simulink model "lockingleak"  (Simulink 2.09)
settings: Solver=ode1  StartTime=0.0  StopTime=1  FixedStep=0.001  MaxStep=0.001  RelTol=1e-5  AbsTol=1e-6

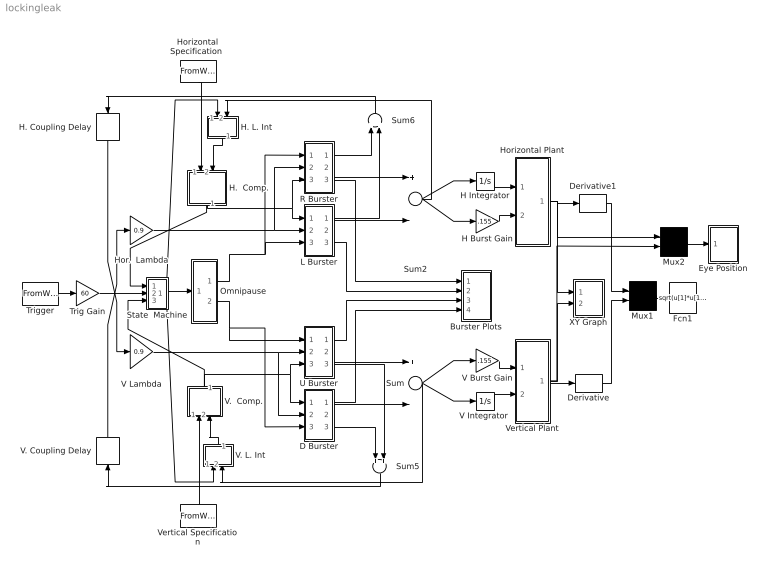
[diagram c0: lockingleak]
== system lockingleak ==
  Burster Plots : Subsystem
  D Burster : Subsystem
  Derivative : Derivative
  Derivative1 : Derivative
  Eye Position : Subsystem  mask(Graph scope.){}
      mask help: Graph scope using MATLAB graph window. Enter plotting ranges and line type.
      mask init:
      | color = @4; ax = [0, @1, @2, @3]; dt = -1;
  Fcn1 : Fcn  Expr=sqrt(u[1]*u[1]+u[2]*u[2])
  H Burst Gain : Gain  Gain=.155
  H Integrator : Integrator  ExternalReset=none  InitialConditionSource=internal  InitialCondition=0  LimitOutput=off  UpperSaturationLimit=inf  LowerSaturationLimit=-inf  ShowSaturationPort=off  ShowStatePort=off  AbsoluteTolerance=auto
  H.  Comp. : Subsystem  Orientation=down
  H. Coupling Delay : TransportDelay  Orientation=down  DelayTime=.001  InitialInput=00  BufferSize=1024
  H. L. Int : Subsystem  Orientation=down
  Hor.  Lambda : Gain  Gain=0.9
  Horizontal Plant : Subsystem
  "Horizontal Specification " : FromWorkspace  Orientation=down  VariableName=hspec
  L Burster : Subsystem
  Mux1 : Mux  Inputs=2
  Mux2 : Mux  Inputs=2
  Omnipause : Subsystem
  R Burster : Subsystem
  State  Machine : Subsystem
  Sum : Sum  Inputs=+-
  Sum2 : Sum  Inputs=+-
  Sum5 : Sum  Orientation=down  Inputs=++
  Sum6 : Sum  Orientation=up  Inputs=++
  Trig Gain : Gain  Gain=60
  Trigger : FromWorkspace  VariableName=trigspec
  U Burster : Subsystem
  V Burst Gain : Gain  Gain=.155
  "V Integrator " : Integrator  ExternalReset=none  InitialConditionSource=internal  InitialCondition=0  LimitOutput=off  UpperSaturationLimit=inf  LowerSaturationLimit=-inf  ShowSaturationPort=off  ShowStatePort=off  AbsoluteTolerance=auto
  V Lambda : Gain  Gain=0.9
  V.  Comp. : Subsystem  Orientation=up
  V. Coupling Delay : TransportDelay  Orientation=up  DelayTime=.001  InitialInput=00  BufferSize=1024
  V. L. Int : Subsystem  Orientation=up
  Vertical Plant : Subsystem
  Vertical Specification : FromWorkspace  Orientation=up  VariableName=vspec
  XY Graph : Subsystem  mask(XY scope.){}
      mask help: XY scope using MATLAB graph window. First input is used as time base. Enter plotting ranges.
      mask init:
      | ax = [@1, @2, @3, @4];st=-1;
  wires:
  State  Machine/1(out_2) -> H. L. Int/1(STATE Input), Omnipause/1(in_1), V. L. Int/1(OPN Input)
  Trig Gain/1 -> State  Machine/2(in_2)
  V.  Comp./1(out_1) -> State  Machine/3(in_3), D Burster/1(in_1), U Burster/3(in_1)
  H.  Comp./1(out_1) -> State  Machine/1(in_1), R Burster/3(in_1), L Burster/1(in_1)
  Omnipause/2(out_4) -> U Burster/1(in_3), D Burster/3(in_3)
  H. L. Int/1(out_1) -> H.  Comp./2(in_2)
  Omnipause/1(out_1) -> R Burster/1(in_3), L Burster/3(in_3)
  Hor.  Lambda/1 -> R Burster/2(in_2), L Burster/2(in_2)
  Mux2/1 -> Eye Position/1(x)
  Horizontal Plant/1(out_1) -> Mux2/1, Derivative1/1, XY Graph/1(x)
  H. Coupling Delay/1 -> V Lambda/1
  V. Coupling Delay/1 -> Hor.  Lambda/1
  Trigger/1 -> Trig Gain/1
  R Burster/1(out_2) -> Sum6/1
  V. L. Int/1(out_1) -> V.  Comp./2(in_5)
  Fcn1/1 -> ?
  Derivative1/1 -> Mux1/1
  Derivative/1 -> Mux1/2
  Mux1/1 -> Fcn1/1
  Vertical Plant/1(out_1) -> Mux2/2, Derivative/1, XY Graph/2(y)
  "Horizontal Specification "/1 -> H.  Comp./1(in_1)
  Vertical Specification/1 -> V.  Comp./1(in_4)
  Sum5/1 -> V. Coupling Delay/1
  Sum6/1 -> H. Coupling Delay/1
  L Burster/1(out_1) -> Sum6/2
  V Lambda/1 -> D Burster/2(in_2), U Burster/2(in_2)
  R Burster/3(out_4) -> Burster Plots/1(in_1)
  L Burster/3(out_3) -> Burster Plots/2(in_2)
  D Burster/1(out_1) -> Burster Plots/4(in_4)
  D Burster/2(out_2) -> Sum/2
  D Burster/3(out_3) -> Sum5/1
  U Burster/1(out_2) -> Burster Plots/3(in_3)
  U Burster/2(out_3) -> Sum/1
  U Burster/3(out_4) -> Sum5/2
  R Burster/2(out_3) -> Sum2/1
  L Burster/2(out_2) -> Sum2/2
  Sum/1 -> V. L. Int/2(BURST Input), "V Integrator "/1, V Burst Gain/1
  "V Integrator "/1 -> Vertical Plant/2(in_2)
  V Burst Gain/1 -> Vertical Plant/1(in_1)
  Sum2/1 -> H. L. Int/2(BURST Input), H Burst Gain/1, H Integrator/1
  H Burst Gain/1 -> Horizontal Plant/2(in_2)
  H Integrator/1 -> Horizontal Plant/1(in_1)

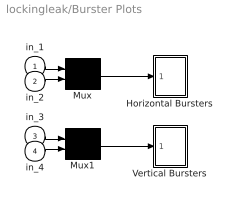
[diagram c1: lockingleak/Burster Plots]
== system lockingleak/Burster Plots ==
  in_1 : Inport  Port=1  PortWidth=-1  SampleTime=-1
  in_2 : Inport  Port=2  PortWidth=-1  SampleTime=-1
  in_3 : Inport  Port=3  PortWidth=-1  SampleTime=-1
  in_4 : Inport  Port=4  PortWidth=-1  SampleTime=-1
  Horizontal Bursters : Subsystem  mask(Graph scope.){}
      mask help: Graph scope using MATLAB graph window. Enter plotting ranges and line type.
      mask init:
      | color = @4; ax = [0, @1, @2, @3]; dt = -1;
  Mux : Mux  Inputs=2
  Mux1 : Mux  Inputs=2
  Vertical Bursters : Subsystem  mask(Graph scope.){}
      mask help: Graph scope using MATLAB graph window. Enter plotting ranges and line type.
      mask init:
      | color = @4; ax = [0, @1, @2, @3]; dt = -1;
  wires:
  in_4/1 -> Mux1/2
  in_3/1 -> Mux1/1
  in_2/1 -> Mux/2
  in_1/1 -> Mux/1
  Mux/1 -> Horizontal Bursters/1(x)
  Mux1/1 -> Vertical Bursters/1(x)

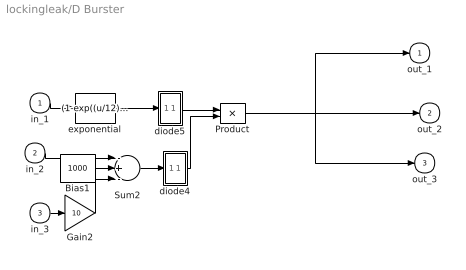
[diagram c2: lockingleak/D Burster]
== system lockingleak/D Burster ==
  in_1 : Inport  Port=1  PortWidth=-1  SampleTime=-1
  in_2 : Inport  Port=2  PortWidth=-1  SampleTime=-1
  in_3 : Inport  Port=3  PortWidth=-1  SampleTime=-1
  Bias1 : Constant  Value=1000
  Gain2 : Gain  Gain=10
  Product : Product  Inputs=2
  Sum2 : Sum  Inputs=-+-
  diode4 : Subsystem
  diode5 : Subsystem
  exponential : Fcn  Expr=(1-exp((u/12)))
  out_1 : Outport  Port=1  InitialOutput=0
  out_2 : Outport  Port=2  InitialOutput=0
  out_3 : Outport  Port=3  InitialOutput=0
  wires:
  in_1/1 -> exponential/1
  Bias1/1 -> Sum2/2
  in_2/1 -> Sum2/1
  in_3/1 -> Gain2/1
  Gain2/1 -> Sum2/3
  Sum2/1 -> diode4/1(in_1)
  diode4/1(out_1) -> Product/2
  exponential/1 -> diode5/1(in_1)
  diode5/1(out_1) -> Product/1
  Product/1 -> out_1/1, out_2/1, out_3/1

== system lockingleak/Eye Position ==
  x : Inport  Port=1  PortWidth=-1  SampleTime=-1
  "S-function M-file which plots lines " : S-Function  FunctionName=sfuny  Parameters=ax, color,dt
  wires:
  x/1 -> "S-function M-file which plots lines "/1

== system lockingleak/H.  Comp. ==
  in_1 : Inport  Port=1  PortWidth=-1  SampleTime=-1
  in_2 : Inport  Port=2  PortWidth=-1  SampleTime=-1
  Sum : Sum  Inputs=+-
  out_1 : Outport  Port=1  InitialOutput=0
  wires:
  in_2/1 -> Sum/2
  in_1/1 -> Sum/1
  Sum/1 -> out_1/1

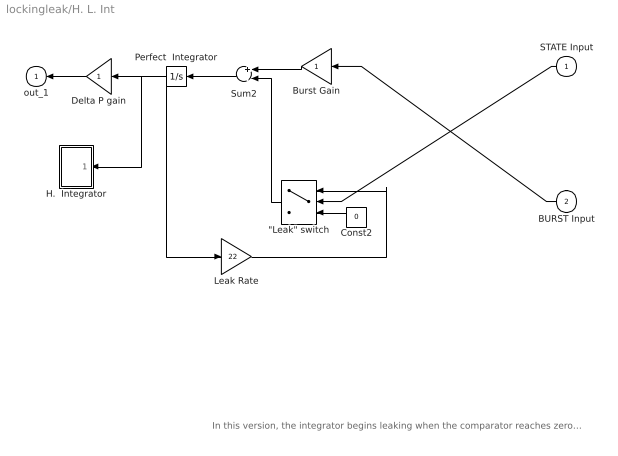
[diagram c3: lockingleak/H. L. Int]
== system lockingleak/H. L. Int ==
  note: In this version, the integrator begins leaking when the comparator reaches zero, and won't stop leaking until either the trigger arrives or the integrator's value goes to zero
  STATE Input : Inport  Orientation=left  Port=1  PortWidth=-1  SampleTime=-1
  BURST Input : Inport  Orientation=left  Port=2  PortWidth=-1  SampleTime=-1
  "\"Leak\" switch" : Switch  Orientation=left  Threshold=0.5
  Burst Gain : Gain  Orientation=left  Gain=1
  Const2 : Constant  Orientation=left  Value=0
  Delta P gain : Gain  Orientation=left  Gain=1
  H.  Integrator : Subsystem  Orientation=left  mask(Graph scope.){}
      mask help: Graph scope using MATLAB graph window. Enter plotting ranges and line type.
      mask init:
      | color = @4; ax = [0, @1, @2, @3]; dt = -1;
  Leak Rate : Gain  Gain=22
  Perfect  Integrator : Integrator  Orientation=left  ExternalReset=none  InitialConditionSource=internal  InitialCondition=0  LimitOutput=off  UpperSaturationLimit=inf  LowerSaturationLimit=-inf  ShowSaturationPort=off  ShowStatePort=off  AbsoluteTolerance=auto
  Sum2 : Sum  Orientation=left  Inputs=+-
  out_1 : Outport  Orientation=left  Port=1  InitialOutput=0
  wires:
  BURST Input/1 -> Burst Gain/1
  STATE Input/1 -> "\"Leak\" switch"/2
  Const2/1 -> "\"Leak\" switch"/3
  "\"Leak\" switch"/1 -> Sum2/2
  Leak Rate/1 -> "\"Leak\" switch"/1
  Perfect  Integrator/1 -> H.  Integrator/1(x), Leak Rate/1, Delta P gain/1
  Burst Gain/1 -> Sum2/1
  Delta P gain/1 -> out_1/1
  Sum2/1 -> Perfect  Integrator/1

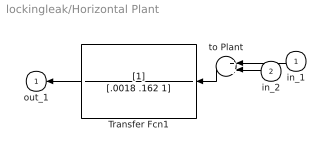
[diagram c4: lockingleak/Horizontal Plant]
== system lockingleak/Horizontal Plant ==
  in_1 : Inport  Orientation=left  Port=1  PortWidth=-1  SampleTime=-1
  in_2 : Inport  Orientation=left  Port=2  PortWidth=-1  SampleTime=-1
  Transfer Fcn1 : TransferFcn  Orientation=left  Numerator=[1]  Denominator=[.0018 .162 1]
  to Plant : Sum  Orientation=left  Inputs=++
  out_1 : Outport  Orientation=left  Port=1  InitialOutput=0
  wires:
  Transfer Fcn1/1 -> out_1/1
  in_2/1 -> to Plant/2
  in_1/1 -> to Plant/1
  to Plant/1 -> Transfer Fcn1/1

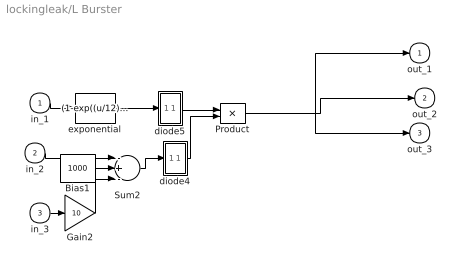
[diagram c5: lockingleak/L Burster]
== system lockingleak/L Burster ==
  in_1 : Inport  Port=1  PortWidth=-1  SampleTime=-1
  in_2 : Inport  Port=2  PortWidth=-1  SampleTime=-1
  in_3 : Inport  Port=3  PortWidth=-1  SampleTime=-1
  Bias1 : Constant  Value=1000
  Gain2 : Gain  Gain=10
  Product : Product  Inputs=2
  Sum2 : Sum  Inputs=-+-
  diode4 : Subsystem
  diode5 : Subsystem
  exponential : Fcn  Expr=(1-exp((u/12)))
  out_1 : Outport  Port=1  InitialOutput=0
  out_2 : Outport  Port=2  InitialOutput=0
  out_3 : Outport  Port=3  InitialOutput=0
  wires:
  Product/1 -> out_3/1, out_2/1, out_1/1
  diode5/1(out_1) -> Product/1
  exponential/1 -> diode5/1(in_1)
  diode4/1(out_1) -> Product/2
  Sum2/1 -> diode4/1(in_1)
  Gain2/1 -> Sum2/3
  in_3/1 -> Gain2/1
  in_2/1 -> Sum2/1
  Bias1/1 -> Sum2/2
  in_1/1 -> exponential/1

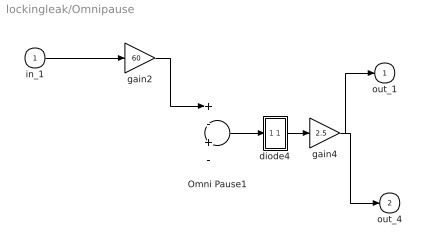
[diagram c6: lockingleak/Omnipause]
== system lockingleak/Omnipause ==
  in_1 : Inport  Port=1  PortWidth=-1  SampleTime=-1
  Omni Pause1 : Sum  Inputs=+-+-
  diode4 : Subsystem
  gain2 : Gain  Gain=60
  gain4 : Gain  Gain=2.5
  out_1 : Outport  Port=1  InitialOutput=0
  out_4 : Outport  Port=2  InitialOutput=0
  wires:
  in_1/1 -> gain2/1
  gain4/1 -> out_4/1, out_1/1
  diode4/1(out_1) -> gain4/1
  gain2/1 -> Omni Pause1/1
  Omni Pause1/1 -> diode4/1(in_1)

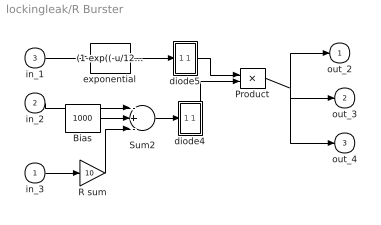
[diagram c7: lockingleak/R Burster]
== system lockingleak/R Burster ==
  in_3 : Inport  Port=1  PortWidth=-1  SampleTime=-1
  in_2 : Inport  Port=2  PortWidth=-1  SampleTime=-1
  in_1 : Inport  Port=3  PortWidth=-1  SampleTime=-1
  Bias : Constant  Value=1000
  Product : Product  Inputs=2
  R sum : Gain  Gain=10
  Sum2 : Sum  Inputs=-+-
  diode4 : Subsystem
  diode5 : Subsystem
  exponential : Fcn  Expr=(1-exp((-u/12)))
  out_2 : Outport  Port=1  InitialOutput=0
  out_3 : Outport  Port=2  InitialOutput=0
  out_4 : Outport  Port=3  InitialOutput=0
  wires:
  diode5/1(out_1) -> Product/1
  exponential/1 -> diode5/1(in_1)
  diode4/1(out_1) -> Product/2
  Sum2/1 -> diode4/1(in_1)
  in_1/1 -> exponential/1
  in_2/1 -> Sum2/1
  Bias/1 -> Sum2/2
  Product/1 -> out_2/1, out_4/1, out_3/1
  in_3/1 -> R sum/1
  R sum/1 -> Sum2/3

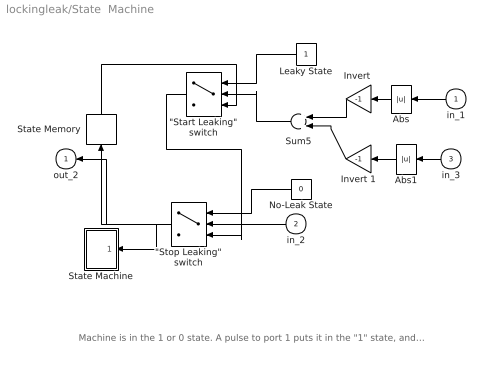
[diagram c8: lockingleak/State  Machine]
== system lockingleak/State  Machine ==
  note: Machine is in the 1 or 0 state. A pulse to port 1 puts it in the "1" state, and a pulse to port 2 puts it in the "0" state.
  in_1 : Inport  Orientation=left  Port=1  PortWidth=-1  SampleTime=-1
  in_2 : Inport  Orientation=left  Port=2  PortWidth=-1  SampleTime=-1
  in_3 : Inport  Orientation=left  Port=3  PortWidth=-1  SampleTime=-1
  "\"Start Leaking\" switch" : Switch  Orientation=left  Threshold=-2
  "\"Stop Leaking\" switch" : Switch  Orientation=left  Threshold=0.001
  Abs : Abs  Orientation=left
  Abs1 : Abs  Orientation=left
  "Invert " : Gain  Orientation=left  Gain=-1
  Invert 1 : Gain  Orientation=left  Gain=-1
  Leaky State : Constant  Orientation=left  Value=1
  No-Leak State : Constant  Orientation=left  Value=0
  State Memory : Memory  Orientation=up  X0=0  InheritSampleTime=off
  State Machine : Subsystem  Orientation=left  mask(Graph scope.){}
      mask help: Graph scope using MATLAB graph window. Enter plotting ranges and line type.
      mask init:
      | color = @4; ax = [0, @1, @2, @3]; dt = -1;
  Sum5 : Sum  Orientation=left  Inputs=++
  out_2 : Outport  Orientation=left  Port=1  InitialOutput=0
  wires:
  Sum5/1 -> "\"Start Leaking\" switch"/2
  "Invert "/1 -> Sum5/1
  Invert 1/1 -> Sum5/2
  Abs1/1 -> Invert 1/1
  in_3/1 -> Abs1/1
  No-Leak State/1 -> "\"Stop Leaking\" switch"/1
  "\"Start Leaking\" switch"/1 -> "\"Stop Leaking\" switch"/3
  Leaky State/1 -> "\"Start Leaking\" switch"/1
  State Memory/1 -> "\"Start Leaking\" switch"/3
  Abs/1 -> "Invert "/1
  "\"Stop Leaking\" switch"/1 -> State Machine/1(x), State Memory/1, out_2/1
  in_1/1 -> Abs/1
  in_2/1 -> "\"Stop Leaking\" switch"/2

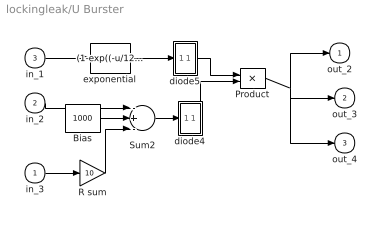
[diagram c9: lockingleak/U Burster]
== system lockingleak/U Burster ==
  in_3 : Inport  Port=1  PortWidth=-1  SampleTime=-1
  in_2 : Inport  Port=2  PortWidth=-1  SampleTime=-1
  in_1 : Inport  Port=3  PortWidth=-1  SampleTime=-1
  Bias : Constant  Value=1000
  Product : Product  Inputs=2
  R sum : Gain  Gain=10
  Sum2 : Sum  Inputs=-+-
  diode4 : Subsystem
  diode5 : Subsystem
  exponential : Fcn  Expr=(1-exp((-u/12)))
  out_2 : Outport  Port=1  InitialOutput=0
  out_3 : Outport  Port=2  InitialOutput=0
  out_4 : Outport  Port=3  InitialOutput=0
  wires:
  diode5/1(out_1) -> Product/1
  exponential/1 -> diode5/1(in_1)
  diode4/1(out_1) -> Product/2
  Sum2/1 -> diode4/1(in_1)
  in_1/1 -> exponential/1
  in_2/1 -> Sum2/1
  Bias/1 -> Sum2/2
  Product/1 -> out_2/1, out_4/1, out_3/1
  in_3/1 -> R sum/1
  R sum/1 -> Sum2/3

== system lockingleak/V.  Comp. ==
  in_4 : Inport  Port=1  PortWidth=-1  SampleTime=-1
  in_5 : Inport  Port=2  PortWidth=-1  SampleTime=-1
  Sum : Sum  Inputs=-+
  out_1 : Outport  Port=1  InitialOutput=0
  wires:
  in_4/1 -> Sum/2
  in_5/1 -> Sum/1
  Sum/1 -> out_1/1

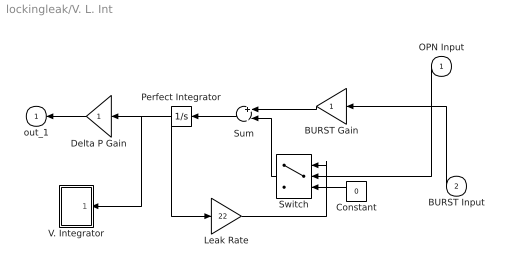
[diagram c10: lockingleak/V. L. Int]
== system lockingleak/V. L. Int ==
  OPN Input : Inport  Orientation=left  Port=1  PortWidth=-1  SampleTime=-1
  BURST Input : Inport  Orientation=left  Port=2  PortWidth=-1  SampleTime=-1
  BURST Gain : Gain  Orientation=left  Gain=1
  Constant : Constant  Orientation=left  Value=0
  Delta P Gain : Gain  Orientation=left  Gain=1
  Leak Rate : Gain  Gain=22
  Perfect Integrator : Integrator  Orientation=left  ExternalReset=none  InitialConditionSource=internal  InitialCondition=0  LimitOutput=off  UpperSaturationLimit=inf  LowerSaturationLimit=-inf  ShowSaturationPort=off  ShowStatePort=off  AbsoluteTolerance=auto
  Sum : Sum  Orientation=left  Inputs=+-
  Switch : Switch  Orientation=left  Threshold=0.5
  V. Integrator : Subsystem  Orientation=left  mask(Graph scope.){}
      mask help: Graph scope using MATLAB graph window. Enter plotting ranges and line type.
      mask init:
      | color = @4; ax = [0, @1, @2, @3]; dt = -1;
  out_1 : Outport  Orientation=left  Port=1  InitialOutput=0
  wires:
  BURST Input/1 -> BURST Gain/1
  OPN Input/1 -> Switch/2
  Sum/1 -> Perfect Integrator/1
  Delta P Gain/1 -> out_1/1
  BURST Gain/1 -> Sum/1
  Perfect Integrator/1 -> Delta P Gain/1, Leak Rate/1, V. Integrator/1(x)
  Leak Rate/1 -> Switch/1
  Constant/1 -> Switch/3
  Switch/1 -> Sum/2

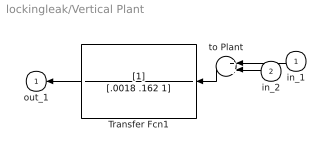
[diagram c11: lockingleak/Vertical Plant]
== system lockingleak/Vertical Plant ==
  in_1 : Inport  Orientation=left  Port=1  PortWidth=-1  SampleTime=-1
  in_2 : Inport  Orientation=left  Port=2  PortWidth=-1  SampleTime=-1
  Transfer Fcn1 : TransferFcn  Orientation=left  Numerator=[1]  Denominator=[.0018 .162 1]
  to Plant : Sum  Orientation=left  Inputs=++
  out_1 : Outport  Orientation=left  Port=1  InitialOutput=0
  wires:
  Transfer Fcn1/1 -> out_1/1
  in_2/1 -> to Plant/2
  in_1/1 -> to Plant/1
  to Plant/1 -> Transfer Fcn1/1

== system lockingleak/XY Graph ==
  x : Inport  Port=1  PortWidth=-1  SampleTime=-1
  y : Inport  Port=2  PortWidth=-1  SampleTime=-1
  Mux : Mux  Inputs=2
  "S-function M-file which plots lines " : S-Function  FunctionName=sfunxy  Parameters=ax, st
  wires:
  Mux/1 -> "S-function M-file which plots lines "/1
  x/1 -> Mux/1
  y/1 -> Mux/2

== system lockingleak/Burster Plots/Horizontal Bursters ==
  x : Inport  Port=1  PortWidth=-1  SampleTime=-1
  "S-function M-file which plots lines " : S-Function  FunctionName=sfuny  Parameters=ax, color,dt
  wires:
  x/1 -> "S-function M-file which plots lines "/1

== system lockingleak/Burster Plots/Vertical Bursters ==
  x : Inport  Port=1  PortWidth=-1  SampleTime=-1
  "S-function M-file which plots lines " : S-Function  FunctionName=sfuny  Parameters=ax, color,dt
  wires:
  x/1 -> "S-function M-file which plots lines "/1

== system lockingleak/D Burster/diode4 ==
  in_1 : Inport  Port=1  PortWidth=-1  SampleTime=-1
  Switch : Switch  Threshold=0
  diode1 : Constant  Value=0
  out_1 : Outport  Port=1  InitialOutput=0
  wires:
  in_1/1 -> Switch/2, Switch/1
  Switch/1 -> out_1/1
  diode1/1 -> Switch/3

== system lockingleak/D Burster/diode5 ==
  in_1 : Inport  Port=1  PortWidth=-1  SampleTime=-1
  Switch : Switch  Threshold=0
  diode1 : Constant  Value=0
  out_1 : Outport  Port=1  InitialOutput=0
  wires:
  in_1/1 -> Switch/2, Switch/1
  Switch/1 -> out_1/1
  diode1/1 -> Switch/3

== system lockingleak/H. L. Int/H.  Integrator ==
  x : Inport  Port=1  PortWidth=-1  SampleTime=-1
  "S-function M-file which plots lines " : S-Function  FunctionName=sfuny  Parameters=ax, color,dt
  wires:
  x/1 -> "S-function M-file which plots lines "/1

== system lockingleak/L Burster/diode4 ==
  in_1 : Inport  Port=1  PortWidth=-1  SampleTime=-1
  Switch : Switch  Threshold=0
  diode1 : Constant  Value=0
  out_1 : Outport  Port=1  InitialOutput=0
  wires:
  diode1/1 -> Switch/3
  Switch/1 -> out_1/1
  in_1/1 -> Switch/2, Switch/1

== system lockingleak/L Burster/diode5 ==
  in_1 : Inport  Port=1  PortWidth=-1  SampleTime=-1
  Switch : Switch  Threshold=0
  diode1 : Constant  Value=0
  out_1 : Outport  Port=1  InitialOutput=0
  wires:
  diode1/1 -> Switch/3
  Switch/1 -> out_1/1
  in_1/1 -> Switch/2, Switch/1

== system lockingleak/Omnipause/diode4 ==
  in_1 : Inport  Port=1  PortWidth=-1  SampleTime=-1
  Switch : Switch  Threshold=0
  diode1 : Constant  Value=0
  out_1 : Outport  Port=1  InitialOutput=0
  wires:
  in_1/1 -> Switch/2, Switch/1
  Switch/1 -> out_1/1
  diode1/1 -> Switch/3

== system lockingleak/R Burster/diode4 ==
  in_1 : Inport  Port=1  PortWidth=-1  SampleTime=-1
  Switch : Switch  Threshold=0
  diode1 : Constant  Value=0
  out_1 : Outport  Port=1  InitialOutput=0
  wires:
  in_1/1 -> Switch/2, Switch/1
  Switch/1 -> out_1/1
  diode1/1 -> Switch/3

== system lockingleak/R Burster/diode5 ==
  in_1 : Inport  Port=1  PortWidth=-1  SampleTime=-1
  Switch : Switch  Threshold=0
  diode1 : Constant  Value=0
  out_1 : Outport  Port=1  InitialOutput=0
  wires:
  diode1/1 -> Switch/3
  Switch/1 -> out_1/1
  in_1/1 -> Switch/2, Switch/1

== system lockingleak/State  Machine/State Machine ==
  x : Inport  Port=1  PortWidth=-1  SampleTime=-1
  "S-function M-file which plots lines " : S-Function  FunctionName=sfuny  Parameters=ax, color,dt
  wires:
  x/1 -> "S-function M-file which plots lines "/1

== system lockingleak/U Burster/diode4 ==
  in_1 : Inport  Port=1  PortWidth=-1  SampleTime=-1
  Switch : Switch  Threshold=0
  diode1 : Constant  Value=0
  out_1 : Outport  Port=1  InitialOutput=0
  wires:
  in_1/1 -> Switch/2, Switch/1
  Switch/1 -> out_1/1
  diode1/1 -> Switch/3

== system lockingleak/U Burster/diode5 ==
  in_1 : Inport  Port=1  PortWidth=-1  SampleTime=-1
  Switch : Switch  Threshold=0
  diode1 : Constant  Value=0
  out_1 : Outport  Port=1  InitialOutput=0
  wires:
  diode1/1 -> Switch/3
  Switch/1 -> out_1/1
  in_1/1 -> Switch/2, Switch/1

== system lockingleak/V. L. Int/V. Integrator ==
  x : Inport  Port=1  PortWidth=-1  SampleTime=-1
  "S-function M-file which plots lines " : S-Function  FunctionName=sfuny  Parameters=ax, color,dt
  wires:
  x/1 -> "S-function M-file which plots lines "/1
